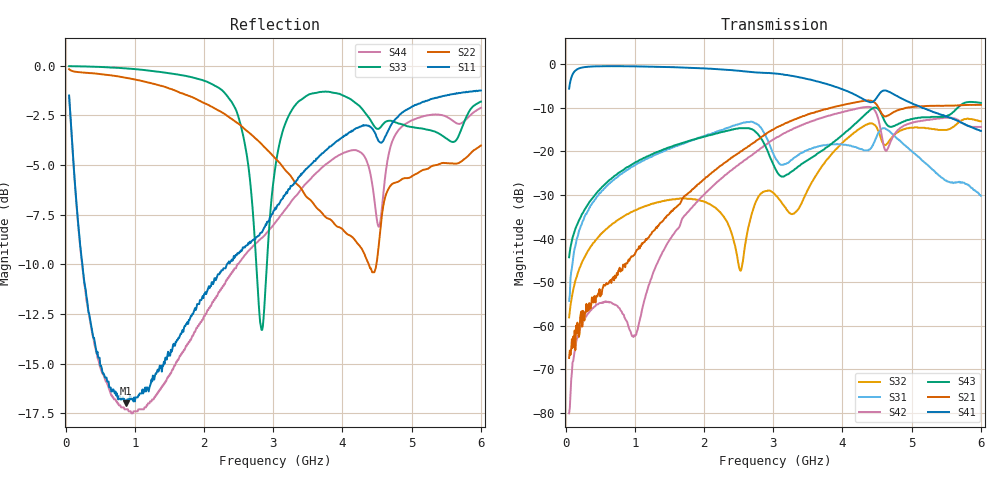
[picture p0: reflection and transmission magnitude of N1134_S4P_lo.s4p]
!S parameter
!Freq	Port1:RFIN1  Port2:RFOUT1  Port3:RFIN2  Port4:RFOUT2
# Hz S dB R 50
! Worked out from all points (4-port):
!   596 points, 50 MHz to 6 GHz, reference 50 ohm
!   strongest paths, dB at 50 MHz, 1.54 GHz, 3.03 GHz, 4.52 GHz, 6 GHz:
!     S41: -5.6, -0.7, -2.2, -7.1, -15.3
!     S21: -67.4, -33.7, -14.7, -10.0, -9.3
!     S43: -44.3, -18.9, -24.0, -10.4, -8.9
!     S42: -80.1, -39.4, -17.0, -12.7, -14.4
!     S31: -54.3, -19.2, -21.5, -15.7, -30.2
!     S32: -58.1, -31.0, -30.0, -15.4, -13.1
!   lowest |S11| = -17.0 dB at 870 MHz (marker M1), VSWR 1.33, Z = 46 - j13.1 ohm
!   |S11| at or under -10 dB: 241.7 MHz to 2.33 GHz (2.088 GHz wide, 162 % of centre)
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5e7  -1.50 -33.6  -68.00 70.1  -54.60 138.0  -5.63 55.9
     -67.40 95.6  -0.18 -2.1  -57.80 82.7  -81.20 45.6
     -54.30 144.0  -58.10 82.7  -0.02 -0.5  -44.30 68.6
     -5.63 56.0  -80.10 32.9  -44.30 68.4  -1.54 -32.3
3e8  -11.60 -79.5  -56.60 97.2  -34.20 94.8  -0.63 7.2
     -55.00 98.2  -0.36 -7.0  -43.40 81.8  -58.00 80.7
     -34.40 95.5  -43.50 81.9  -0.04 -3.1  -32.70 72.8
     -0.63 7.2  -57.80 80.5  -32.70 72.8  -11.80 -71.7
8.7e8  -17.00 -99.0  -45.90 145.0  -24.50 70.8  -0.49 -15.5
       -45.70 145.0  -0.61 -20.0  -34.60 72.9  -58.50 32.5
       -24.50 71.2  -34.60 72.9  -0.14 -10.1  -23.80 73.1
       -0.49 -15.5  -58.70 32.6  -23.80 73.1  -17.30 -85.5
2.52e9  -9.39 -157.0  -20.20 159.0  -13.90 -4.1  -1.55 -61.3
        -20.10 159.0  -2.98 -75.8  -48.60 87.1  -22.80 179.0
        -13.70 -2.7  -47.30 78.2  -2.86 -56.8  -14.70 29.4
        -1.54 -61.3  -22.80 179.0  -14.70 30.0  -9.85 -156.0
3.14e9  -6.68 -175.0  -13.90 136.0  -22.10 -29.7  -2.40 -79.9
        -13.90 136.0  -5.10 -109.0  -32.00 90.9  -16.00 146.0
        -23.10 -31.3  -32.20 91.3  -3.25 -2.8  -25.70 28.5
        -2.34 -79.7  -16.00 146.0  -25.80 28.9  -7.40 -178.0
4.31e9  -3.02 141.0  -8.42 74.2  -19.70 -37.5  -8.12 -108.0
        -8.42 74.1  -9.42 167.0  -14.20 108.0  -9.88 60.3
        -19.80 -37.1  -14.20 108.0  -2.29 -77.5  -11.90 77.9
        -8.13 -108.0  -9.89 60.2  -11.80 78.4  -4.53 132.0
6e9  -1.25 121.0  -9.38 37.4  -30.10 -76.0  -15.30 -131.0
     -9.35 37.2  -4.02 122.0  -13.20 39.8  -14.30 25.9
     -30.20 -74.3  -13.10 39.9  -1.81 160.0  -8.90 39.8
     -15.30 -130.0  -14.40 25.9  -8.89 39.8  -2.12 119.0
